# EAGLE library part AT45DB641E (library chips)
64 Mbit flash memory
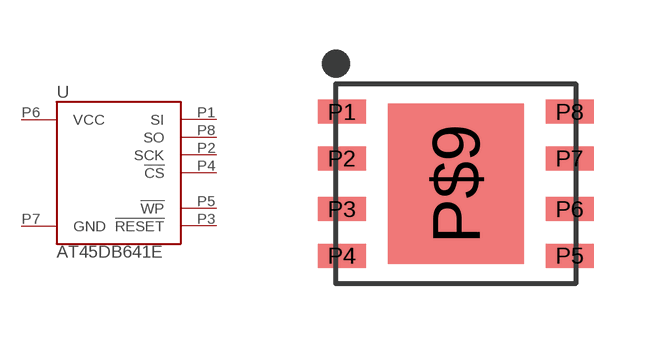
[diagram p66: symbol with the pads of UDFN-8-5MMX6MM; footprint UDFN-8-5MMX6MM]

Designator prefix U

## AT45DB641EUDFN (DIGIKEY: AT45DB641E-MHN-TCT-ND; MANUFACTURER: Adesto; MPN: AT45DB641E-MHN-T)  [UDFN-8-5MMX6MM]
P1  SI
P2  SCK
P3  !RESET
P4  !CS
P5  !WP
P6  VCC
P7  GND
P8  SO

## Footprint UDFN-8-5MMX6MM (pad centres in mm)
smd 1.2 x 0.6: P1 -2.85,1.8; P2 -2.85,0.635; P3 -2.85,-0.635; P4 -2.85,-1.8; P5 2.85,-1.8; P6 2.85,-0.635; P7 2.85,0.635; P8 2.85,1.8
smd 3.4 x 4: P$9 0,0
